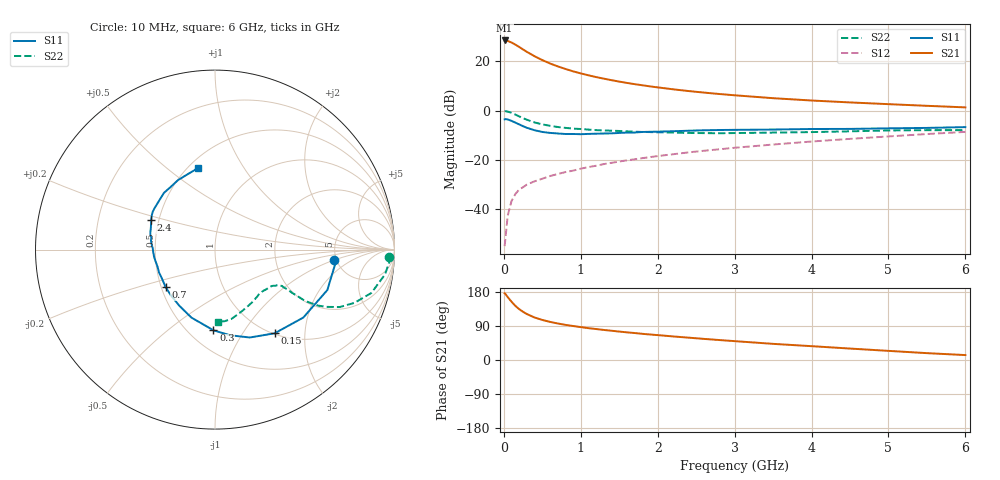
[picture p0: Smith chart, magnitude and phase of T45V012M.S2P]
! Infineon Technologies  Discrete & RF Semiconductors
! BFR182T
! Si NPN RF Bipolar Junction Transistor in SC75
! VCE = 5 V  IC = 12 mA
! Common Emitter S-Parameters:  October  1999
# GHz  S  MA  R  50
!  f  S11  S21  S12  S22
! GHz  MAG  ANG  MAG  ANG  MAG  ANG  MAG  ANG
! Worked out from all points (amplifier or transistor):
!   36 points, 10 MHz to 6 GHz, reference 50 ohm
!   highest |S21| = 28.4 dB at 10 MHz (marker M1)
!   |S21| within 3 dB of that: start of sweep to 217.7 MHz
!   unconditionally stable (mu >= 1): 928.7 MHz to 3.792 GHz
!   at 250 MHz: K = 0.49, MSG = 27.9 dB, |S12| = -31.0 dB
!   at 1.4 GHz: K = 1.07, MAG = 15.1 dB, |S12| = -21.1 dB
!   at 6 GHz: K = 0.85, MSG = 5.0 dB, |S12| = -8.6 dB
!   S11 on the Smith chart (normalised r, x): 10 MHz: 4.78, -1.02; 150 MHz: 1.01, -1.41; 300 MHz: 0.65, -0.74; 700 MHz: 0.53, -0.25; 2.4 GHz: 0.45, +0.18; 6 GHz: 0.56, +0.65
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0.01  0.667 -5.1  26.44 175.9  0.0018 79.9  0.9697 -2.4
0.02  0.675 -6.6  26.4 174.4  0.0025 96.6  0.9769 -3.3
0.05  0.6652 -19.8  25.82 166.0  0.0074 83.9  0.9575 -8.3
0.1  0.6208 -37.6  24.03 153.8  0.0148 74.4  0.904 -15.5
0.15  0.5726 -54.5  21.78 142.8  0.0205 68.5  0.8317 -20.9
0.2  0.5268 -68.4  19.51 134.1  0.0253 65.8  0.7657 -24.7
0.25  0.4844 -80.1  17.35 127.1  0.0282 62.6  0.7032 -27.0
0.3  0.4496 -91.1  15.51 121.2  0.0319 60.9  0.6545 -28.5
0.4  0.4011 -109.1  12.66 112.1  0.0371 60.1  0.5768 -29.7
0.5  0.3705 -122.5  10.59 105.7  0.0418 60.5  0.528 -29.4
0.6  0.3544 -133.7  9.037 100.6  0.0474 61.3  0.4932 -29.3
0.7  0.3454 -142.9  7.895 96.4  0.052 62.5  0.4669 -28.9
0.9  0.3371 -157.8  6.267 89.7  0.061 64.9  0.433 -28.7
1.1  0.3382 -169.5  5.202 84.0  0.072 65.2  0.4134 -29.0
1.3  0.3447 -177.8  4.45 79.3  0.0828 66.3  0.3976 -30.0
1.6  0.3604 172.0  3.648 73.0  0.0987 66.9  0.3808 -32.0
2.2  0.3829 158.6  2.708 62.2  0.131 67.2  0.3601 -38.2
2.4  0.3922 155.1  2.499 59.0  0.1429 67.0  0.3535 -40.6
3.5  0.4145 138.2  1.79 42.6  0.206 63.6  0.3596 -55.1
4.5  0.4272 125.6  1.469 30.2  0.2684 59.1  0.3813 -69.8
5.5  0.4475 109.5  1.254 18.1  0.3361 53.6  0.4027 -82.4
6  0.4644 101.6  1.166 13.0  0.3716 50.0  0.4029 -87.4
